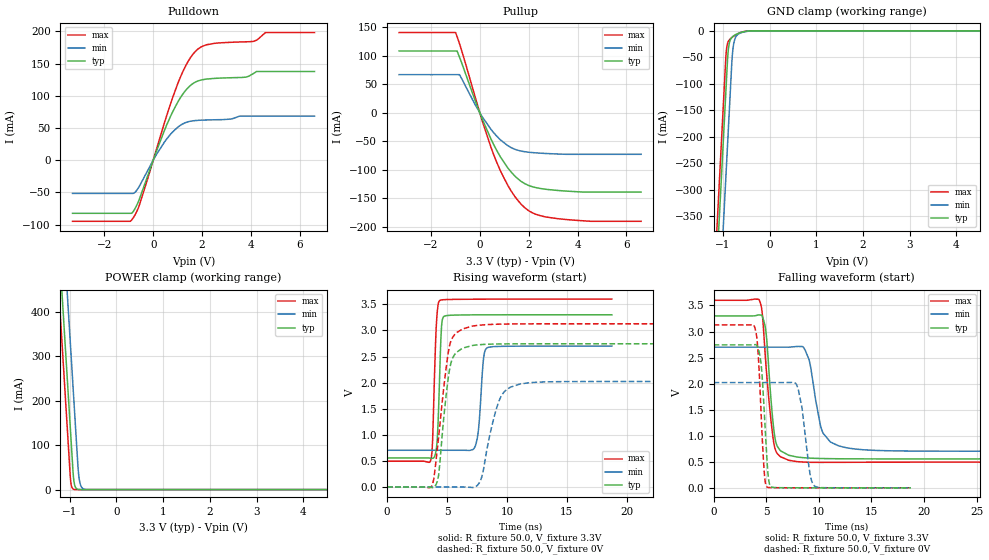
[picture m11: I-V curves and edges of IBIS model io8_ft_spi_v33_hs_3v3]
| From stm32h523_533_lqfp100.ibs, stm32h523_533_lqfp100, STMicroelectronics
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[Model]   io8_ft_spi_v33_hs_3v3
Model_type I/O
Polarity   Non-Inverting
Enable   Active-Low
| CAP_THRESHOLD on pad IOFT is "UDTCAPC" :
| Rising=20.0% of vddiom   Falling=80.0% of vddiom
| C_comp min and max val. don't necessarily correlate with the min and max pvt
| but are the smallest and greatest pad capacitance found.
| var   typ   min   max
C_comp   3.95307pF  3.95031pF  4.00762pF
|C_comp_pullup   2.45745pF  2.54015pF  2.38930pF
|C_comp_pulldown   1.49562pF  1.41016pF  1.61832pF
Vinl = 810.0mV
Vinh = 2.52V
Vmeas = 1.65V   | Reference voltage for timing measurements
Cref  = 50.0pF   | Timing specification test load capacitance value
Rref  = 100.0MOhm   | Timing specification test load resistance value
Vref  = 1.65V   | Timing specification test load voltage
[Model Spec]
| TIME_THRESHOLD on pin ZIV33M is "CMOS" :
| Rising=40.0% of vddiom   Falling=60.0% of vddiom
Vinl 1.28680V 1.06380V 1.39380V
Vinh 1.76920V 1.48820V 1.89120V
| variable   typ   min   max
[Temperature Range] 25.0 125.0 -40.0
| variable   typ   min   max
[Voltage Range] 3.3V 2.7V 3.6V
| variable   typ   min   max
[POWER Clamp Reference] 3.3V 2.7V 3.6V
| variable   typ   min   max
[GND Clamp Reference] 0V 0V 0V
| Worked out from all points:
|   slope of the pulldown table from 0 to 0.495 V, typ, clamps not added: 10 ohm
|   slope of the pullup table from 0 to 0.495 V, typ, clamps not added: 10 ohm
|   GND clamp passes 1 mA (typ) near -0.52 V on its own axis
|   POWER clamp passes 1 mA (typ) near -0.84 V on its own axis
|   rising waveform, R_fixture 50.0, V_fixture 3.3V: 20-80 % time 245ps typ, 358ps min, 255ps max; typ from 0.556 V to 3.3 V
|   falling waveform, R_fixture 50.0, V_fixture 3.3V: 20-80 % time 645ps typ, 1.06ns min, 789ps max; typ from 3.3 V to 0.556 V
|   rising waveform, R_fixture 50.0, V_fixture 0V: 20-80 % time 738ps typ, 1.19ns min, 914ps max; typ from 0 V to 2.74 V
|   falling waveform, R_fixture 50.0, V_fixture 0V: 20-80 % time 477ps typ, 738ps min, 455ps max; typ from 2.74 V to 0 V
[POWER Clamp]
-3.3V     4.068A     4.259A     3.957A
-1.25V    582.8mA    774.2mA    471.5mA
-1.21V    514.8mA    706.2mA    403.5mA
-1.13V    378.8mA    570.2mA    267.5mA
-1.04V    225.8mA    417.2mA    114.5mA
-980mV    123.8mA    315.2mA    17.95mA
-920mV    26.3mA     213.2mA    906uA
-880mV    5.543mA    145.2mA    123.7uA
-810mV    363.5uA    33.6mA     3.798uA
-770mV    76.62uA    10.47mA    519.4nA
-690mV    3.409uA    1.017mA    10.48nA
6.6V      0A         0A         0A
[GND Clamp]
-3.3V     -4.13A     -4.291A    -4.063A
-1.25V    -644.7mA   -806.4mA   -578.1mA
-940mV    -117.7mA   -279.4mA   -51.06mA
-920mV    -83.75mA   -245.4mA   -31.43mA
-900mV    -50.5mA    -211.4mA   -23.14mA
-880mV    -31.27mA   -177.4mA   -19.1mA
-850mV    -18.68mA   -126.4mA   -15.73mA
-800mV    -11.46mA   -46.4mA    -12.03mA
-760mV    -8.752mA   -20.02mA   -9.606mA
-680mV    -5.122mA   -6.673mA   -5.579mA
-320mV    -10.25uA   -73.91uA   -1.981uA
6.6V      10.49nA    1.843uA    393.6pA
| variable   typ   min   max
[Pullup Reference] 3.3V 2.7V 3.6V
| variable   typ   min   max
[Pulldown Reference] 0V 0V 0V
[Pullup]
-3.3V     108.7mA    67.06mA    141mA
-990mV    108.7mA    67.06mA    141mA
-930mV    108.7mA    67.06mA    133.9mA
-830mV    97.78mA    67.06mA    121.3mA
120mV     -12.97mA   -8.371mA   -17mA
680mV     -65.16mA   -40.47mA   -85.72mA
1.3V      -105mA     -61.6mA    -138.6mA
1.64V     -119mA     -66.82mA   -158.3mA
1.97V     -127.3mA   -69.18mA   -171.3mA
2.51V     -133.3mA   -71.08mA   -181.3mA
3.4V      -137.3mA   -72.8mA    -187.1mA
6.6V      -139.3mA   -72.98mA   -190.8mA
[Pulldown]
-3.3V     -82.42mA   -51.49mA   -94.82mA
-850mV    -81.27mA   -51.49mA   -91.26mA
-580mV    -62.01mA   -41.36mA   -71.41mA
120mV     12.61mA    7.999mA    15.37mA
800mV     75.3mA     43.94mA    97.52mA
1.33V     108.3mA    58.37mA    146.5mA
1.84V     123.1mA    61.83mA    172.7mA
2.51V     126.9mA    62.7mA     181.3mA
3.78V     128.8mA    68.32mA    183.7mA
4.12V     134.9mA    68.32mA    184.6mA
4.59V     137.6mA    68.32mA    198mA
6.6V      137.6mA    68.32mA    198mA
[Ramp]
dV/dt_r 1.64651V/735.9435ps 1.21266V/1.18941ns 1.87653V/911.66762ps
dV/dt_f 1.64666V/643.32846ps 1.19801V/1.05739ns 1.86387V/788.72113ps
R_load = 50.0
| Removed startup time: 0s 0s 0s  .
| Removed end time: 18.75ns.
[Rising Waveform]
R_fixture   = 50.0
V_fixture   = 3.3V
V_fixture_min = 2.7V
V_fixture_max = 3.6V
0s        555.6mV    703.3mV    493.6mV
3.65ns    551.1mV    703.3mV    517.3mV
3.8ns     549.5mV    703.3mV    893.9mV
4.15ns    806.6mV    703.3mV    3.246V
4.4ns     2.217V     703.3mV    3.574V
4.55ns    3.092V     703.3mV    3.585V
4.7ns     3.258V     703.3mV    3.589V
7.3ns     3.299V     756.3mV    3.598V
8.35ns    3.299V     2.667V     3.599V
18.75ns   3.3V       2.7V       3.6V
| Removed startup time: 0s 0s 0s  .
| Removed end time: 38.75ns.
[Falling Waveform]
R_fixture   = 50.0
V_fixture   = 3.3V
V_fixture_min = 2.7V
V_fixture_max = 3.6V
0s        3.3V       2.7V       3.6V
4.35ns    3.319V     2.7V       3.598V
4.6ns     3.304V     2.7V       3.385V
4.95ns    3.026V     2.7V       2.415V
5.75ns    1.067V     2.7V       826.5mV
7.15ns    625mV      2.7V       528.8mV
8.7ns     576.3mV    2.642V     493.9mV
10.3ns    563mV      1.099V     488.8mV
11.9ns    558.5mV    804.7mV    489.8mV
38.75ns   555.6mV    703.3mV    493.6mV
| Removed startup time: 0s 0s 0s  .
| Removed end time: 38.6ns.
[Rising Waveform]
R_fixture   = 50.0
V_fixture   = 0V
V_fixture_min = 0V
V_fixture_max = 0V
0s        228.5nV    416.9nV    212.6nV
3.8ns     -13.71mV   445nV      51.95mV
4.3ns     219.7mV    430.4nV    954mV
4.8ns     1.485V     649.7nV    2.041V
5.2ns     2.232V     2.142uV    2.695V
6.3ns     2.66V      160.1uV    3.028V
7.7ns     2.726V     81.21mV    3.1V
9.4ns     2.741V     1.683V     3.12V
11.1ns    2.743V     1.973V     3.125V
38.6ns    2.744V     2.021V     3.128V
| Removed startup time: 0s 0s 0s  .
| Removed end time: 18.75ns.
[Falling Waveform]
R_fixture   = 50.0
V_fixture   = 0V
V_fixture_min = 0V
V_fixture_max = 0V
0s        2.744V     2.021V     3.128V
3.9ns     2.748V     2.021V     3.084V
4.2ns     2.697V     2.021V     2.667V
4.5ns     2.392V     2.021V     1.477V
4.8ns     1.498V     2.021V     332mV
5.05ns    603mV      2.021V     20.76mV
5.4ns     28.35mV    2.021V     4.91mV
7.9ns     1.447mV    1.971V     1.212mV
9.6ns     679.8uV    30.37mV    707.9uV
18.75ns   16.32uV    177.8uV    21.16uV
